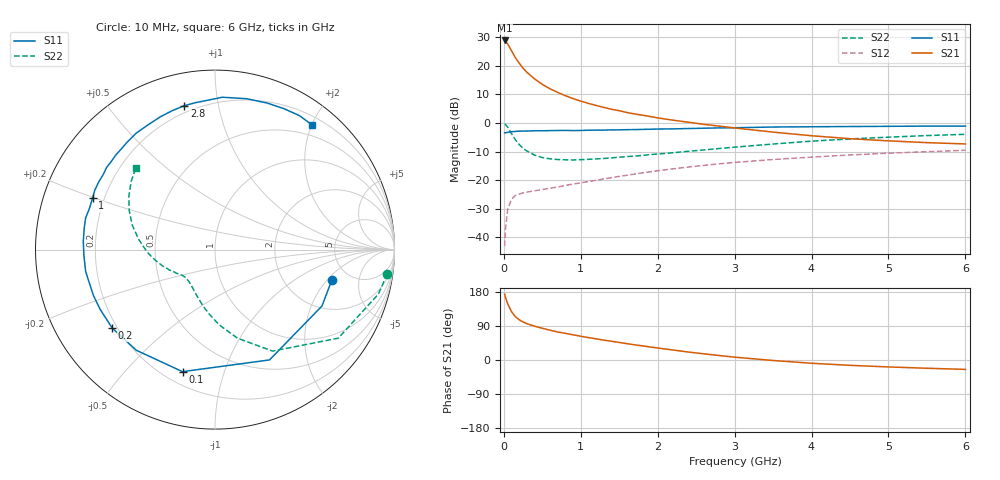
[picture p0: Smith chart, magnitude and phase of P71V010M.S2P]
! SIEMENS Small Signal Semiconductors
! BFP196
! Si NPN RF Bipolar Junction Transistor in SOT143
! VCE = 1 V  IC = 10 mA
! Common Emitter S-Parameters:  May  1996
# GHz  S  MA  R  50
!  f  S11  S21  S12  S22
! GHz  MAG  ANG  MAG  ANG  MAG  ANG  MAG  ANG
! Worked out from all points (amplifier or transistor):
!   36 points, 10 MHz to 6 GHz, reference 50 ohm
!   highest |S21| = 28.9 dB at 10 MHz (marker M1)
!   |S21| within 3 dB of that: start of sweep to 87.26 MHz
!   unconditionally stable (mu >= 1): 857.1 MHz to 5.19 GHz; 5.715 GHz to end of sweep
!   at 250 MHz: K = 0.41, MSG = 21.8 dB, |S12| = -24.5 dB
!   at 1.4 GHz: K = 1.15, MAG = 9.6 dB, |S12| = -19.2 dB
!   at 6 GHz: K = 1.01, MAG = 0.6 dB, |S12| = -9.6 dB
!   S11 on the Smith chart (normalised r, x): 10 MHz: 3.67, -2.24; 100 MHz: 0.27, -0.73; 200 MHz: 0.18, -0.33; 1 GHz: 0.16, +0.20; 2.8 GHz: 0.16, +0.80; 6 GHz: 0.32, +2.00
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0.01  0.6729 -14.4  27.77 173.9  0.007 85.4  0.969 -8.0
0.02  0.6738 -27.8  26.82 166.0  0.0136 76.4  0.9437 -15.2
0.05  0.6856 -63.7  24.15 148.2  0.031 61.9  0.8457 -35.7
0.1  0.7036 -104.9  18.33 127.3  0.0464 45.3  0.6504 -60.4
0.15  0.7119 -128.0  13.9 114.4  0.0538 36.7  0.5097 -75.7
0.2  0.7204 -142.6  11.11 106.2  0.0569 32.6  0.4195 -86.9
0.25  0.7213 -152.5  9.065 100.2  0.0599 30.6  0.3595 -95.3
0.3  0.724 -159.3  7.698 95.9  0.0617 29.9  0.3234 -101.6
0.4  0.7308 -170.3  5.901 89.2  0.0652 30.3  0.2739 -112.1
0.5  0.7311 -177.3  4.739 83.7  0.0683 31.4  0.2485 -119.7
0.6  0.7353 176.3  3.968 78.7  0.0722 33.0  0.2361 -125.1
0.7  0.7385 170.4  3.423 74.0  0.076 34.5  0.2296 -129.5
0.8  0.7421 166.3  2.999 70.3  0.0806 35.8  0.2269 -133.3
1  0.7401 157.2  2.414 62.7  0.0897 38.6  0.2282 -138.9
1.1  0.7473 153.6  2.203 59.1  0.0945 39.5  0.2314 -141.1
1.6  0.7638 136.2  1.525 43.1  0.1218 41.2  0.2581 -150.8
2.2  0.7887 118.3  1.119 26.3  0.1577 38.9  0.3017 -161.6
2.8  0.8198 102.0  0.882 11.8  0.1931 33.7  0.3577 -174.1
3.5  0.8499 87.2  0.692 -1.3  0.2295 26.2  0.4284 172.5
4.5  0.8669 70.3  0.531 -14.1  0.2759 15.1  0.5259 155.4
5.5  0.8822 57.9  0.453 -21.8  0.315 4.1  0.6022 140.9
6  0.8807 52.3  0.43 -24.8  0.3327 -2.0  0.6341 134.0
